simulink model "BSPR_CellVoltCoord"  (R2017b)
settings: Solver=FixedStepDiscrete  StartTime=0.0  StopTime=10.0  FixedStep=0.02  RelTol=1e-3  EnableMultiTasking=on
undefined symbols (not defined in the file): bin2dec, BSPR_CellVoltVldChkDisbl_C, BSPR_cntCellInvldNum_C, BSPR_cntCellSerNum_C, BSPR_cntCellVoltOutRngDiag_CW, BSPR_cntCellVoltVldDiag_CW, BSPR_cntCellVoltVldHi_C, BSPR_cntVoltCellAvl_C, BSPR_iCellVoltDeltaBattCurr_X, BSPR_rCellVoltDeltaBattSOC_Y, BSPR_tBattTempForCellHi_C, BSPR_tBattTempForCellLo_C, BSPR_tiCellVoltInvldChk_C, BSPR_tiCellVoltInvldChkdT_C, BSPR_tiCellVoltRngHiChk_C, BSPR_tiCellVoltRngHiChkdT_C, BSPR_tiCellVoltRngLoChk_C, BSPR_tiCellVoltRngLoChkdT_C, BSPR_uCellVoltDelta_Z, BSPR_uCellVoltHi_C, BSPR_uCellVoltLo_C, BSPR_uCellVoltMaxLim_C, BSPR_uCellVoltMinLim_C
libraries: simulink x35, AIWAYS_Powertrain_BMS_lib x2
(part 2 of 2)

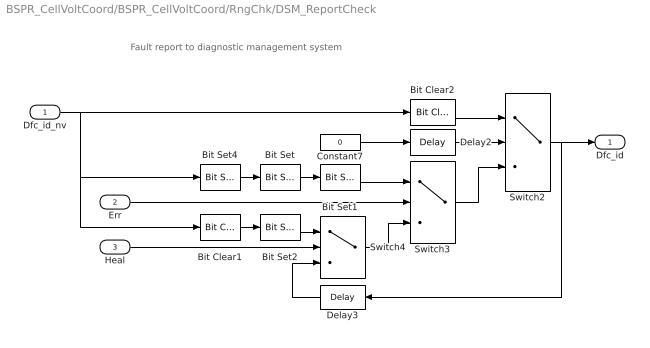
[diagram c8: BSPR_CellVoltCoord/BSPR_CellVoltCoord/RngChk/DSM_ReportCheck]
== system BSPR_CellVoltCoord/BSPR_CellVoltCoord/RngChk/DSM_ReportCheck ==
  note: Fault report to diagnostic management system
  Dfc_id_nv : Inport  OutDataTypeStr=uint8
  Err : Inport  Port=2
  Heal : Inport  Port=3
  Bit Clear1 : simulink/Logic and Bit Operations/Bit Clear  iBit=4
  Bit Clear2 : simulink/Logic and Bit Operations/Bit Clear  iBit=3
  Bit Set : simulink/Logic and Bit Operations/Bit Set  iBit=4
  Bit Set1 : simulink/Logic and Bit Operations/Bit Set  iBit=3
  Bit Set2 : simulink/Logic and Bit Operations/Bit Set  iBit=3
  Bit Set4 : simulink/Logic and Bit Operations/Bit Set  iBit=7
  Constant7 : Constant  Value=0  OutDataTypeStr=boolean
  Delay2 : Delay  DelayLength=1  InitialCondition=1
  Delay3 : Delay  DelayLength=1  InitialCondition=0
  Switch2 : Switch  Criteria=u2 ~= 0
  Switch3 : Switch  Criteria=u2 ~= 0
  Switch4 : Switch  Criteria=u2 ~= 0
  Dfc_id : Outport  OutDataTypeStr=uint8
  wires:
  Dfc_id_nv/1 -> Bit Clear2/1, Bit Set4/1, Bit Clear1/1
  Bit Set4/1 -> Bit Set/1
  Constant7/1 -> Delay2/1
  Delay2/1 -> Switch2/2
  Switch3/1 -> Switch2/3
  Bit Clear2/1 -> Switch2/1
  Switch2/1 -> Delay3/1, Dfc_id/1
  Bit Set1/1 -> Switch3/1
  Bit Set/1 -> Bit Set1/1
  Switch4/1 -> Switch3/3
  Err/1 -> Switch3/2
  Bit Set2/1 -> Switch4/1
  Bit Clear1/1 -> Bit Set2/1
  Delay3/1 -> Switch4/3
  Heal/1 -> Switch4/2

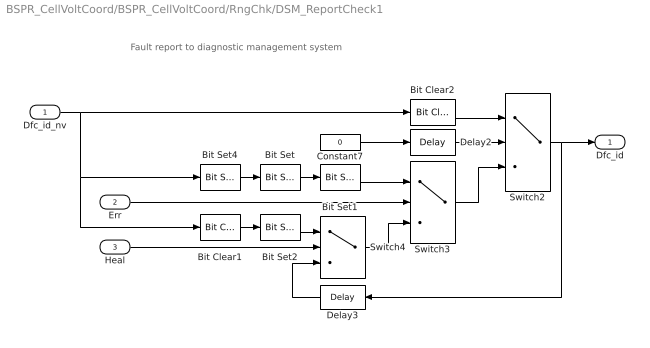
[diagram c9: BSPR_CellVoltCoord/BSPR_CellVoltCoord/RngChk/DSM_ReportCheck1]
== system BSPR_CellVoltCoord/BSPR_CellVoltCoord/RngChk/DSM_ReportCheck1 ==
  note: Fault report to diagnostic management system
  Dfc_id_nv : Inport  OutDataTypeStr=uint8
  Err : Inport  Port=2
  Heal : Inport  Port=3
  Bit Clear1 : simulink/Logic and Bit Operations/Bit Clear  iBit=4
  Bit Clear2 : simulink/Logic and Bit Operations/Bit Clear  iBit=3
  Bit Set : simulink/Logic and Bit Operations/Bit Set  iBit=4
  Bit Set1 : simulink/Logic and Bit Operations/Bit Set  iBit=3
  Bit Set2 : simulink/Logic and Bit Operations/Bit Set  iBit=3
  Bit Set4 : simulink/Logic and Bit Operations/Bit Set  iBit=7
  Constant7 : Constant  Value=0  OutDataTypeStr=boolean
  Delay2 : Delay  DelayLength=1  InitialCondition=1
  Delay3 : Delay  DelayLength=1  InitialCondition=0
  Switch2 : Switch  Criteria=u2 ~= 0
  Switch3 : Switch  Criteria=u2 ~= 0
  Switch4 : Switch  Criteria=u2 ~= 0
  Dfc_id : Outport  OutDataTypeStr=uint8
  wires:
  Heal/1 -> Switch4/2
  Delay3/1 -> Switch4/3
  Bit Clear1/1 -> Bit Set2/1
  Bit Set2/1 -> Switch4/1
  Err/1 -> Switch3/2
  Switch4/1 -> Switch3/3
  Bit Set/1 -> Bit Set1/1
  Bit Set1/1 -> Switch3/1
  Switch2/1 -> Dfc_id/1, Delay3/1
  Bit Clear2/1 -> Switch2/1
  Switch3/1 -> Switch2/3
  Delay2/1 -> Switch2/2
  Constant7/1 -> Delay2/1
  Bit Set4/1 -> Bit Set/1
  Dfc_id_nv/1 -> Bit Clear1/1, Bit Set4/1, Bit Clear2/1

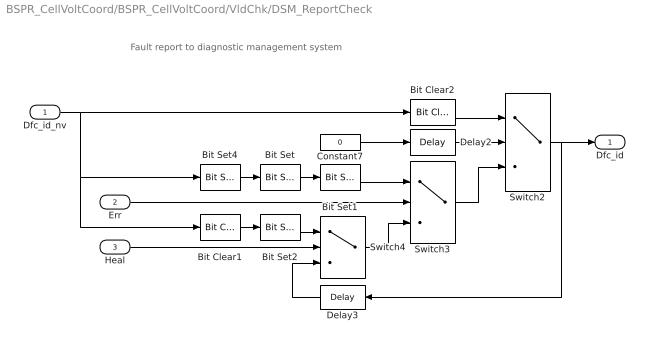
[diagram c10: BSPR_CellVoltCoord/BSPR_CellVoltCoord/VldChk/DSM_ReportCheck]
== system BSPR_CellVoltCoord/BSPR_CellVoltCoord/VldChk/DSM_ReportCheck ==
  note: Fault report to diagnostic management system
  Dfc_id_nv : Inport  OutDataTypeStr=uint8
  Err : Inport  Port=2
  Heal : Inport  Port=3
  Bit Clear1 : simulink/Logic and Bit Operations/Bit Clear  iBit=4
  Bit Clear2 : simulink/Logic and Bit Operations/Bit Clear  iBit=3
  Bit Set : simulink/Logic and Bit Operations/Bit Set  iBit=4
  Bit Set1 : simulink/Logic and Bit Operations/Bit Set  iBit=3
  Bit Set2 : simulink/Logic and Bit Operations/Bit Set  iBit=3
  Bit Set4 : simulink/Logic and Bit Operations/Bit Set  iBit=7
  Constant7 : Constant  Value=0  OutDataTypeStr=boolean
  Delay2 : Delay  DelayLength=1  InitialCondition=1
  Delay3 : Delay  DelayLength=1  InitialCondition=0
  Switch2 : Switch  Criteria=u2 ~= 0
  Switch3 : Switch  Criteria=u2 ~= 0
  Switch4 : Switch  Criteria=u2 ~= 0
  Dfc_id : Outport  OutDataTypeStr=uint8
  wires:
  Dfc_id_nv/1 -> Bit Clear2/1, Bit Set4/1, Bit Clear1/1
  Bit Set4/1 -> Bit Set/1
  Constant7/1 -> Delay2/1
  Delay2/1 -> Switch2/2
  Switch3/1 -> Switch2/3
  Bit Clear2/1 -> Switch2/1
  Switch2/1 -> Delay3/1, Dfc_id/1
  Bit Set1/1 -> Switch3/1
  Bit Set/1 -> Bit Set1/1
  Switch4/1 -> Switch3/3
  Err/1 -> Switch3/2
  Bit Set2/1 -> Switch4/1
  Bit Clear1/1 -> Bit Set2/1
  Delay3/1 -> Switch4/3
  Heal/1 -> Switch4/2

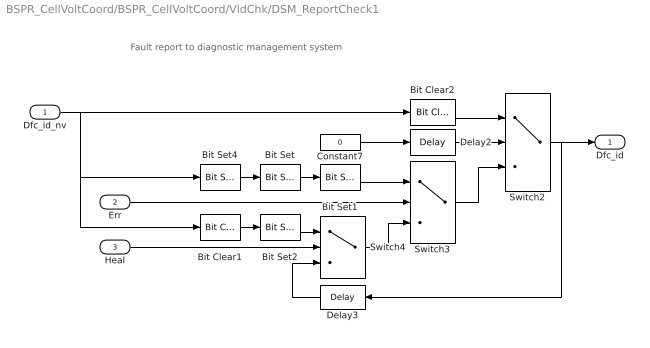
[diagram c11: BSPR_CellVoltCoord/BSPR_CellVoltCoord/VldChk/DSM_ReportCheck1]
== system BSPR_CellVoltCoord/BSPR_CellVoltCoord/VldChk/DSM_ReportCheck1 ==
  note: Fault report to diagnostic management system
  Dfc_id_nv : Inport  OutDataTypeStr=uint8
  Err : Inport  Port=2
  Heal : Inport  Port=3
  Bit Clear1 : simulink/Logic and Bit Operations/Bit Clear  iBit=4
  Bit Clear2 : simulink/Logic and Bit Operations/Bit Clear  iBit=3
  Bit Set : simulink/Logic and Bit Operations/Bit Set  iBit=4
  Bit Set1 : simulink/Logic and Bit Operations/Bit Set  iBit=3
  Bit Set2 : simulink/Logic and Bit Operations/Bit Set  iBit=3
  Bit Set4 : simulink/Logic and Bit Operations/Bit Set  iBit=7
  Constant7 : Constant  Value=0  OutDataTypeStr=boolean
  Delay2 : Delay  DelayLength=1  InitialCondition=1
  Delay3 : Delay  DelayLength=1  InitialCondition=0
  Switch2 : Switch  Criteria=u2 ~= 0
  Switch3 : Switch  Criteria=u2 ~= 0
  Switch4 : Switch  Criteria=u2 ~= 0
  Dfc_id : Outport  OutDataTypeStr=uint8
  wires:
  Heal/1 -> Switch4/2
  Delay3/1 -> Switch4/3
  Bit Clear1/1 -> Bit Set2/1
  Bit Set2/1 -> Switch4/1
  Err/1 -> Switch3/2
  Switch4/1 -> Switch3/3
  Bit Set/1 -> Bit Set1/1
  Bit Set1/1 -> Switch3/1
  Switch2/1 -> Dfc_id/1, Delay3/1
  Bit Clear2/1 -> Switch2/1
  Switch3/1 -> Switch2/3
  Delay2/1 -> Switch2/2
  Constant7/1 -> Delay2/1
  Bit Set4/1 -> Bit Set/1
  Dfc_id_nv/1 -> Bit Clear1/1, Bit Set4/1, Bit Clear2/1

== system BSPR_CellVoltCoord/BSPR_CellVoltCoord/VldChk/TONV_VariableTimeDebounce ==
  note: Turn On Delay Time Deboune
  u : Inport
  T : Inport  Port=2
  dT : Inport  Port=3
  Add : Sum
  Constant1 : Constant  Value=0  OutDataTypeStr=single
  Constant2 : Constant  OutDataTypeStr=uint8
  Constant3 : Constant  Value=0  OutDataTypeStr=uint8
  Delay : Delay  DelayLength=1  InitialCondition=0
  MinMax : MinMax  Inputs=2
  Product : Product  OutMin=[0]  OutMax=[65535]  OutDataTypeStr=single
  Relational Operator : RelationalOperator  Operator=>  OutDataTypeStr=boolean  RndMeth=Simplest
  Switch : Switch  Criteria=u2 ~= 0
  Switch1 : Switch  Criteria=u2 ~= 0
  y : Outport
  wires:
  Switch1/1 -> Product/1
  Constant3/1 -> Switch1/3
  Constant2/1 -> Switch1/1
  u/1 -> Switch1/2, Switch/2
  dT/1 -> Switch/1
  Constant1/1 -> Switch/3
  Add/1 -> Product/2
  Product/1 -> Relational Operator/1, Delay/1
  Switch/1 -> Add/1
  Delay/1 -> MinMax/2
  Relational Operator/1 -> y/1
  T/1 -> MinMax/1, Relational Operator/2
  MinMax/1 -> Add/2

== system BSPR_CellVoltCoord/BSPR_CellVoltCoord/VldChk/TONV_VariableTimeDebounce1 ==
  note: Turn On Delay Time Deboune
  u : Inport
  T : Inport  Port=2
  dT : Inport  Port=3
  Add : Sum
  Constant1 : Constant  Value=0  OutDataTypeStr=single
  Constant2 : Constant  OutDataTypeStr=uint8
  Constant3 : Constant  Value=0  OutDataTypeStr=uint8
  Delay : Delay  DelayLength=1  InitialCondition=0
  MinMax : MinMax  Inputs=2
  Product : Product  OutMin=[0]  OutMax=[65535]  OutDataTypeStr=single
  Relational Operator : RelationalOperator  Operator=>  OutDataTypeStr=boolean  RndMeth=Simplest
  Switch : Switch  Criteria=u2 ~= 0
  Switch1 : Switch  Criteria=u2 ~= 0
  y : Outport
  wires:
  Switch1/1 -> Product/1
  Constant3/1 -> Switch1/3
  Constant2/1 -> Switch1/1
  u/1 -> Switch1/2, Switch/2
  dT/1 -> Switch/1
  Constant1/1 -> Switch/3
  Add/1 -> Product/2
  Product/1 -> Relational Operator/1, Delay/1
  Switch/1 -> Add/1
  Delay/1 -> MinMax/2
  Relational Operator/1 -> y/1
  T/1 -> MinMax/1, Relational Operator/2
  MinMax/1 -> Add/2

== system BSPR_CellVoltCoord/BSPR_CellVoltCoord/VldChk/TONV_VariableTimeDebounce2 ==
  note: Turn On Delay Time Deboune
  u : Inport
  T : Inport  Port=2
  dT : Inport  Port=3
  Add : Sum
  Constant1 : Constant  Value=0  OutDataTypeStr=single
  Constant2 : Constant  OutDataTypeStr=uint8
  Constant3 : Constant  Value=0  OutDataTypeStr=uint8
  Delay : Delay  DelayLength=1  InitialCondition=0
  MinMax : MinMax  Inputs=2
  Product : Product  OutMin=[0]  OutMax=[65535]  OutDataTypeStr=single
  Relational Operator : RelationalOperator  Operator=>  OutDataTypeStr=boolean  RndMeth=Simplest
  Switch : Switch  Criteria=u2 ~= 0
  Switch1 : Switch  Criteria=u2 ~= 0
  y : Outport
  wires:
  MinMax/1 -> Add/2
  T/1 -> Relational Operator/2, MinMax/1
  Relational Operator/1 -> y/1
  Delay/1 -> MinMax/2
  Switch/1 -> Add/1
  Product/1 -> Delay/1, Relational Operator/1
  Add/1 -> Product/2
  Constant1/1 -> Switch/3
  dT/1 -> Switch/1
  u/1 -> Switch/2, Switch1/2
  Constant2/1 -> Switch1/1
  Constant3/1 -> Switch1/3
  Switch1/1 -> Product/1

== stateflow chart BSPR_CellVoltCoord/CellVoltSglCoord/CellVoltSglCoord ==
  state SglCoord_Stt
    (default) -> (junction 10) : % SglCoord
    (junction 9) -> (junction 27) : [GaBSW_CellVoltVld_flg[i]==boolean(1)]
    (junction 11) -> (junction 9) : [i<BSPR_cntCellVoltSmpl_C]
    (junction 10) -> (junction 11) : {i=0;}
    (junction 9) -> (junction 12) : {BSPR_uCellVolt_A[i]=BSPR_uCellVoltAvrg;}
    (junction 27) -> (junction 37) : {BSPR_uCellVolt_A[i]=COMR_uCellVolt_A[i]/1000;}
    (junction 12) -> (junction 11) : {i = i + 1;}
    (junction 11) -> (junction 13)
    (junction 37) -> (junction 12)
  (default) -> SglCoord_Stt
  (junction 25) -> SglCoord_Stt
  (junction 23) -> (junction 25)
  SglCoord_Stt -> (junction 21)
  (junction 21) -> (junction 23)
  data: COMR_uCellVolt_A input; BSPR_uCellVoltAvrg input; GaBSW_CellVoltVld_flg input; i local uint8; BSPR_cntCellVoltSmpl_C input; BSPR_uCellVolt_A output

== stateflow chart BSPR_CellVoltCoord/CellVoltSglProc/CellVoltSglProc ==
  state SglProc_Stt
    (default) -> (junction 10) : %SglProc
    (junction 9) -> (junction 27) : [GaBSW_CellVoltVld_flg[i]==boolean(1)||... BSPR_CellVoltVldChkDisbl_C]
    (junction 27) -> (junction 37) : {BSPR_uSumVoltCellAvl=BSPR_uSumVoltCellAvl+COMR_uCellVolt_A[i]; BSPR_cntVoltCellAvl=BSPR_cntVoltCellAvl+1; BSPR_bCellVoltInvld_A[i]=0;}
    (junction 37) -> (junction 53) : [COMR_uCellVolt_A[i] < BSPR_uCellVoltMinTmp]
    (junction 11) -> (junction 9) : [i<BSPR_cntCellSerNum_C]
    (junction 10) -> (junction 11) : {i=0; BSPR_uSumVoltCellAvl=0; BSPR_cntVoltCellAvl=0; BSPR_uCellVoltMinTmp=5000; BSPR_uCellVoltMaxTmp=0;}
    (junction 9) -> (junction 12) : {BSPR_bCellVoltInvld_A[i]=1;}
    (junction 37) -> (junction 54)
    (junction 53) -> (junction 55) : {BSPR_uCellVoltMinTmp=COMR_uCellVolt_A[i]; BSPR_idxCellVoltMin=i+1;}
    (junction 55) -> (junction 54)
    (junction 54) -> (junction 61)
    (junction 12) -> (junction 11) : {i = i + 1;}
    (junction 11) -> (junction 13)
    (junction 61) -> (junction 60) : [COMR_uCellVolt_A[i] > BSPR_uCellVoltMaxTmp]
    (junction 61) -> (junction 57)
    (junction 60) -> (junction 58) : {BSPR_uCellVoltMaxTmp=COMR_uCellVolt_A[i]; BSPR_idxCellVoltMax=i+1;}
    (junction 57) -> (junction 12)
    (junction 58) -> (junction 57)
  (default) -> SglProc_Stt
  (junction 25) -> SglProc_Stt
  (junction 23) -> (junction 25)
  SglProc_Stt -> (junction 21)
  (junction 21) -> (junction 23)
  data: COMR_uCellVolt_A input; GaBSW_CellVoltVld_flg input boolean; BSPR_CellVoltVldChkDisbl_C input; BSPR_uSumVoltCellAvl output single; BSPR_cntCellSerNum_C input; i local uint8; BSPR_cntVoltCellAvl output uint8; BSPR_uCellVoltMaxTmp output single; BSPR_uCellVoltMinTmp output single; BSPR_idxCellVoltMax output; BSPR_idxCellVoltMin output; BSPR_bCellVoltInvld_A output
